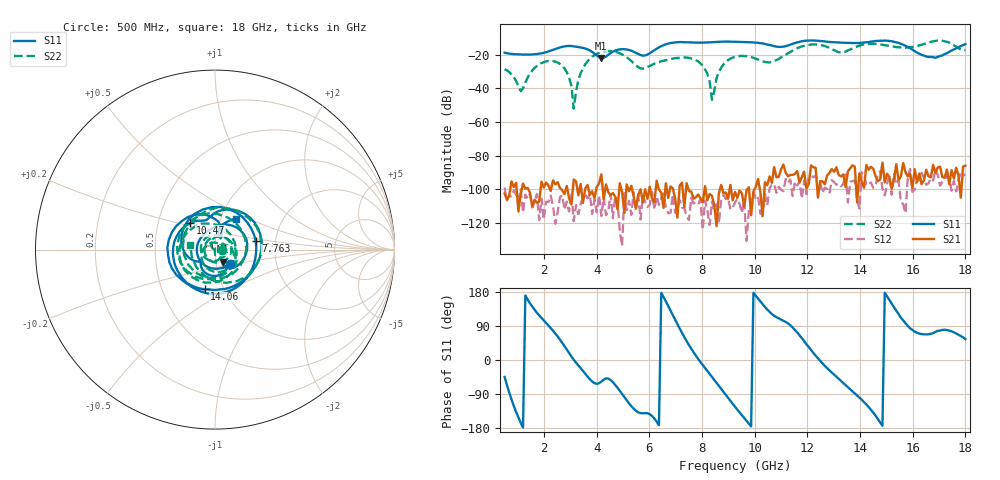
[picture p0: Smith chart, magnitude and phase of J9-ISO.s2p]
!Agilent Technologies,N5230A,MY45001360,A.07.50.67
!Agilent N5230A: A.07.50.67
!Date: Tuesday, April 16, 2024 16:07:12
!Correction: S11(Full 2 Port(1,2))
!S21(Full 2 Port(1,2))
!S12(Full 2 Port(1,2))
!S22(Full 2 Port(1,2))
!S2P File: Measurements: S11, S21, S12, S22:
# Hz S  dB  R 50
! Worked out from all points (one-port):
!   201 points, 500 MHz to 18 GHz, reference 50 ohm
!   lowest |S11| = -22.0 dB at 4.175 GHz (marker M1), VSWR 1.17, Z = 54 - j7.28 ohm
!   |S11| at or under -10 dB: start of sweep to end of sweep
!   S11 on the Smith chart (normalised r, x): 500 MHz: 1.16, -0.19; 7.763 GHz: 1.58, +0.16; 10.47 GHz: 0.73, +0.22; 14.06 GHz: 0.81, -0.38; 18 GHz: 1.19, +0.42
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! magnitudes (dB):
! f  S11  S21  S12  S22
! 500 MHz  -18.7  -102.6  -99.1  -28.6
! 1.113 GHz  -19.8  -102.7  -100.2  -41.7
! 1.725 GHz  -19.5  -108.1  -103.0  -26.7
! 2.513 GHz  -16.1  -95.9  -113.9  -24.6
! 2.95 GHz  -14.7  -105.5  -113.3  -33.5
! 3.125 GHz  -14.9  -94.3  -119.1  -52.1
! 3.3 GHz  -15.4  -103.7  -114.9  -35.2
! 3.475 GHz  -15.9  -108.2  -105.0  -28.1
! 4.175 GHz  -22.0  -91.2  -116.0  -18.4
! 5.662 GHz  -20.1  -100.1  -118.1  -28.1
! 6.362 GHz  -15.5  -100.4  -109.5  -24.3
! 7.763 GHz  -12.7  -104.9  -107.9  -23.2
! 8.2 GHz  -12.6  -106.6  -112.6  -31.3
! 8.375 GHz  -12.5  -104.0  -107.5  -46.8
! 8.637 GHz  -12.2  -102.6  -120.6  -30.1
! 9.25 GHz  -12.2  -101.7  -107.9  -21.2
! 10.47 GHz  -13.8  -97.7  -109.6  -24.4
! 12.22 GHz  -11.5  -86.9  -93.0  -13.8
! 14.06 GHz  -12.8  -95.7  -90.0  -14.1
! 15.11 GHz  -11.7  -92.8  -91.6  -14.7
! 16.86 GHz  -21.8  -90.4  -88.4  -11.8
! 18 GHz  -13.7  -86.0  -92.0  -17.1
